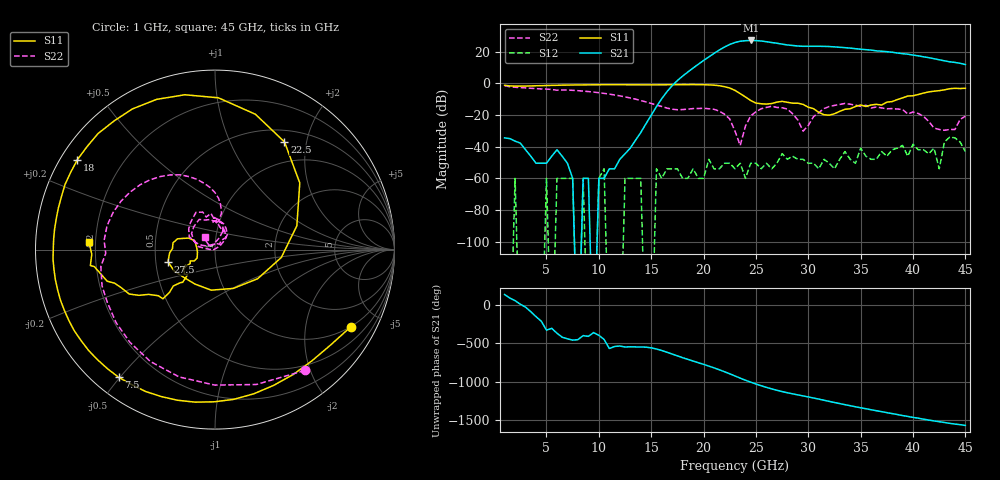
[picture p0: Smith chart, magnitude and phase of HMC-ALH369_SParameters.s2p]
! Analog Devices, Inc.
! Device:	HMC-ALH369
! Description:	GaAs HEMT MMIC LOW NOISE AMPLIFIER, 24 - 40 GHz
! Conditions:	Vdd = 5.0 V
!		Vgg = OPEN
!		Operating Temperature = +25 C
! Freq(GHz)	S11a(dB)	S11p(deg)	S21a(dB)	S21p(deg)	S12a(dB)	S12p(deg)	S22a(dB)	S22p(deg)
# GHz S DB R 50
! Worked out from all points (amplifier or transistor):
!   89 points, 1 GHz to 45 GHz, reference 50 ohm
!   highest |S21| = 27.1 dB at 24.5 GHz (marker M1)
!   |S21| within 3 dB of that: 22.35 GHz to 28.24 GHz (5.892 GHz wide, 23.3 % of centre)
!   unconditionally stable (mu >= 1): start of sweep to end of sweep
!   at 8 GHz: K = 65557376171024968.00, MAG = -120.0 dB, |S12| = -180.0 dB
!   at 23 GHz: K = 8.18, MAG = 27.8 dB, |S12| = -54.0 dB
!   at 45 GHz: K = 9.15, MAG = 14.9 dB, |S12| = -43.1 dB
!   S11 on the Smith chart (normalised r, x): 1 GHz: 0.99, -3.52; 7.5 GHz: 0.07, -0.50; 18 GHz: 0.05, +0.30; 22.5 GHz: 0.67, +1.63; 27.5 GHz: 0.58, -0.09; 45 GHz: 0.17, +0.03
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1  -1.21 -29.7  -34.42 130.1  -180.00 -4.2  -1.52 -53.4
7.5  -1.00 -127.0  -60.00 -100.2  -60.00 134.8  -4.38 159.9
8.5  -0.94 -136.8  -60.00 -41.3  -60.00 15.9  -4.87 145.8
16  -0.89 165.2  -9.68 126.1  -60.00 -116.4  -14.56 80.8
18  -0.76 146.8  4.61 33.0  -60.00 152.7  -16.54 93.4
20.5  -0.93 111.2  16.74 -76.0  -47.96 139.6  -16.03 78.2
21.5  -1.45 88.8  21.08 -123.4  -53.98 168.9  -17.52 62.1
22.5  -2.93 57.2  24.62 -176.0  -50.46 -168.5  -22.50 44.0
23  -4.42 38.2  25.84 156.1  -53.98 108.6  -30.17 36.1
24  -8.59 -6.8  26.99 101.1  -60.00 169.8  -26.94 174.4
24.5  -10.81 -34.3  27.14 76.2  -50.46 130.7  -20.54 169.7
25.5  -12.88 -95.3  26.78 29.6  -53.98 116.7  -16.03 145.8
26  -13.07 -120.0  26.34 8.7  -50.46 59.9  -15.19 132.7
27.5  -11.34 -165.4  24.80 -45.8  -44.44 150.1  -15.39 100.0
29  -12.51 170.8  23.61 -88.6  -47.96 69.7  -23.10 69.6
30.5  -15.97 156.3  23.45 -129.1  -50.46 -19.5  -21.01 162.6
32.5  -19.17 -154.8  23.09 172.7  -53.98 15.5  -13.89 133.0
34.5  -14.61 -150.0  21.94 117.7  -50.46 96.4  -13.76 106.6
36  -13.64 -146.9  21.04 78.7  -47.96 38.1  -15.55 91.1
38  -11.50 -136.2  19.72 29.3  -41.94 52.7  -15.92 84.3
41.5  -5.38 -152.6  16.27 -54.5  -44.44 -32.7  -24.01 55.7
45  -3.06 176.6  11.93 -124.3  -43.10 -110.7  -20.72 128.2
